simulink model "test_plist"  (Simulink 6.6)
settings: Solver=ode45  StartTime=0.0  StopTime=10.0  RelTol=1e-3
libraries: sltpda x4

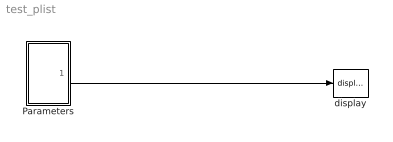
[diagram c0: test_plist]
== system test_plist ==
  Parameters : Subsystem
  display : sltpda/AO class/display  Tag=display  SystemSampleTime=-1
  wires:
  Parameters/1(Out1) -> display/1

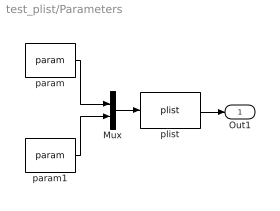
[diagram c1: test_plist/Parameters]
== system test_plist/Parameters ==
  Mux : Mux  Inputs=2
  param : sltpda/AO class/Parameters/param  Tag=param  SystemSampleTime=-1  key=a  value=1
  param1 : sltpda/AO class/Parameters/param  Tag=param  SystemSampleTime=-1  key=b  value=2
  plist : sltpda/AO class/Parameters/plist  SystemSampleTime=-1
  Out1 : Outport
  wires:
  param/1 -> Mux/1
  param1/1 -> Mux/2
  Mux/1 -> plist/1
  plist/1 -> Out1/1
